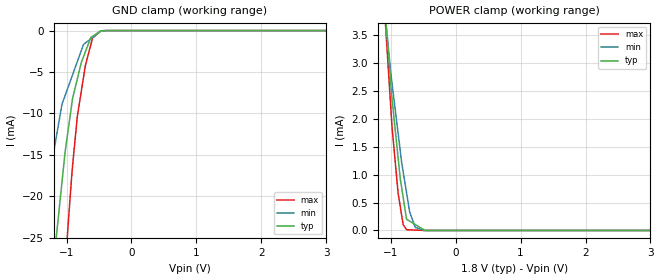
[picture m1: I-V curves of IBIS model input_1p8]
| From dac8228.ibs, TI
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|   input_1p8 Model
[Model]   input_1p8
Model_type   Input
Vinl = 0.3
Vinh = 1.5
|   typ   min   max
|   (nom PVT)   (Fast PVT)   (slow PVT)
|C_comp from frequency method(F=50MHz)
|Average
|C_comp   4.965e-12   4.262e-12   5.457e-12
|C_comp from L-C Tank method(L=1nH)
|Resonant Frequency(Hz)   2.85e9   2.855e9   2.81e9
C_comp   3.122e-12   3.121e-12   3.211e-12
| Where nom  PVT is Nominal Process,  1.8V,  33C
|   Fast PVT is Strong Process,   1.89V,  -40C
|   Slow PVT is Weak Process,   1.71V,  113C
[Voltage Range]   1.8   1.71   1.89
|Ambient Temperature   25   105   -40
|Junction Temperature
[Temperature Range]   33   113   -40
[Power Clamp Reference]   1.8   1.71   1.89
[GND Clamp Reference]   0   0   0
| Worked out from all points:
|   GND clamp passes 1 mA (typ) near -0.63 V on its own axis
|   POWER clamp passes 1 mA (typ) near -0.86 V on its own axis
[GND Clamp]
|   Voltage   I(typ)   I(min)   I(max)
-1.8V     -88.66mA   -48.53mA   -133.7mA
-1.366V   -43.56mA   -22.25mA   -73.59mA
-1.175V   -26.27mA   -13.65mA   -47.78mA
-1.07V    -18.32mA   -8.928mA   -34.43mA
-1.021V   -14.58mA   -7.819mA   -28.44mA
-929.9mV  -9.488mA   -5.843mA   -18.55mA
-907.2mV  -8.214mA   -5.349mA   -16.33mA
-833.5mV  -5.831mA   -3.743mA   -10.35mA
-710.6mV  -2.585mA   -1.508mA   -4.264mA
-599.1mV  -698.5uA   -834.4uA   -901.3uA
-471.6mV  -31.07uA   -64.03uA   -35.72uA
3.6V      0A         0A         0A
[POWER Clamp]
|   Voltage   I(typ)   I(min)   I(max)
-1.8V     17.37mA    14.7mA     20.61mA
-1.079V   3.836mA    3.784mA    3.674mA
-977.1mV  2.334mA    2.613mA    1.828mA
-886.4mV  1.308mA    1.747mA    674.3uA
-853.2mV  933.1uA    1.429mA    431.6uA
-831.1mV  766.5uA    1.218mA    269.8uA
-808.9mV  599.9uA    1.058mA    108uA
-756mV    201.7uA    677uA      13.91uA
-707.9mV  167.7uA    333.9uA    11.57uA
-622.4mV  107uA      56.17uA    7.402uA
-470.3mV  14.94nA    738.6nA    0A
3.6V      0A         0A         0A
